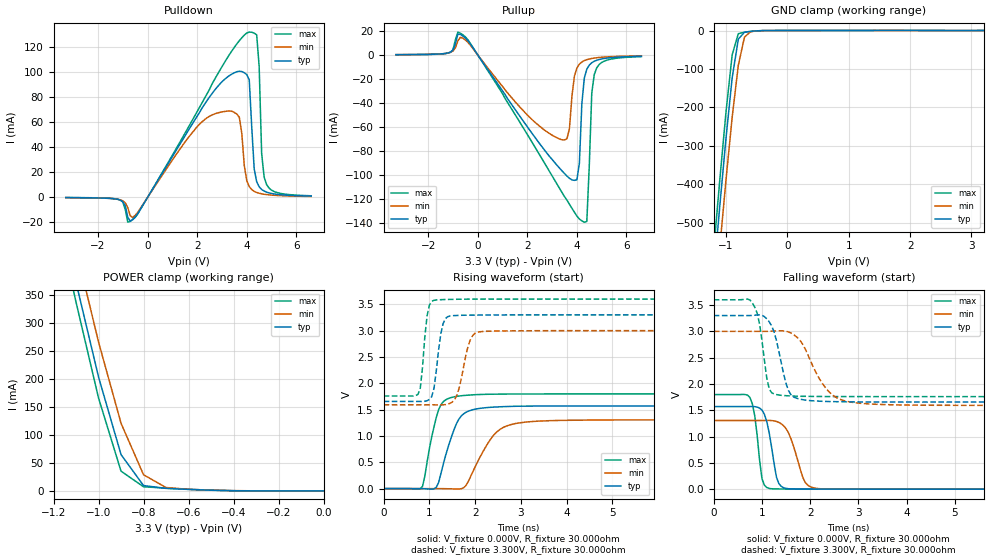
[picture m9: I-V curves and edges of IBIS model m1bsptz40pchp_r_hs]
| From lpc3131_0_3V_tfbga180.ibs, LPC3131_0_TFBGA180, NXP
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| |   Rev 0.20 IBIS Model Design Automation Generation   |
| |   N O N - S I L I C O N   C O R R E L A T E D   |
| |   This IBIS [Model] is pre-Beta tactical support   |
| |  Note: this IBIS [Model] contains clamp curves generated   |
| |   through simulation which should not be relied upon   |
| Date/Time   : 2010 Jan 25 (Mon) 11:58:19
| Pccmos090 jliolib_p50 2.0
|   0.9 um 3.3V pad library
|   seven level metal
|   dual oxide
|   dual threshold voltage
|   nominal line mixed supply
|   parasitic extracted netlists
| Process block a10
| mem1bsptz40pchp
|   Bidirectional Pad 3.3
|   3state Output
|   Plain Input
|   CMOS
|   Programmable between
|   - (p1=0, p2=1) plain input
|   - (p1=0, p2=0) with Pull Up
|   - (p1=1, p2=1) with Pull Down
|   - (p1=1, p2=0) with Repeater
| Repeater Mode high speed(esh=0, p1=1, p2=0)
[Model]   m1bsptz40pchp_r_hs | of mem1bsptz40pchp
Model_type   I/O
Polarity   Non-Inverting
Enable   Active-Low
|  Reciever Thresholds
Vinl   = 0.99V
Vinh   = 2.31V
| AC Test Load Conditions
Vref   = 0
Cref   = 0
Rref   = 1000000000
Vmeas   = 1.65
| [Process Range]   typical   min   max
| C_comp edge width   400.000ps   400.000ps   400.000ps
| C_comp Tstrobe   40.000fs   40.000fs   40.000fs
C_comp   200.000pF   200.000pF   200.000pF
[Temperature Range]   25   125   -40
[Voltage Range]   3.30V   3.00V   3.60V
[GND Clamp Reference]   0.00V   0.00V   0.00V
[Pulldown Reference]   0.00V   0.00V   0.00V
[POWER Clamp Reference]   3.30V   3.00V   3.60V
[Pullup Reference]   3.30V   3.00V   3.60V
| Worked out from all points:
|   slope of the pulldown table from 0 to 0.495 V, typ, clamps not added: 30.9 ohm
|   slope of the pullup table from 0 to 0.495 V, typ, clamps not added: 33.4 ohm
|   GND clamp passes 1 mA (typ) near -0.51 V on its own axis
|   POWER clamp passes 1 mA (typ) near -0.47 V on its own axis
|   rising waveform, V_fixture 0.000V, R_fixture 30.000ohm: 20-80 % time 345ps typ, 518ps min, 258ps max; typ from 0 V to 1.57 V
|   falling waveform, V_fixture 0.000V, R_fixture 30.000ohm: 20-80 % time 178ps typ, 273ps min, 137ps max; typ from 1.57 V to 0 V
|   rising waveform, V_fixture 3.300V, R_fixture 30.000ohm: 20-80 % time 145ps typ, 213ps min, 116ps max; typ from 1.66 V to 3.3 V
|   falling waveform, V_fixture 3.300V, R_fixture 30.000ohm: 20-80 % time 251ps typ, 503ps min, 170ps max; typ from 3.3 V to 1.66 V
[GND Clamp]
| ref voltage   0.00V   0.00V   0.00V
|   Voltage   I(typ)   I(min)   I(max)
-3.3V     -4.732A    -4.814A    -4.684A
-1.2V     -636mA     -742.5mA   -569.7mA
-1.1V     -453.5mA   -561.8mA   -385.7mA
-1V       -279mA     -387.5mA   -210.8mA
-900mV    -122.8mA   -225.5mA   -63.13mA
-800mV    -22.45mA   -90.49mA   -8.204mA
-700mV    -4.394mA   -17.31mA   -4.534mA
-600mV    -2.163mA   -3.055mA   -2.529mA
-300mV    -78.17uA   -69.01uA   -98.11uA
3.2V      -17.82uA   34.39uA    -87.56uA
[Power Clamp]   | Vtable = Vcc - Vpad
| ref voltage   3.30V   3.00V   3.60V
|   Voltage   I(typ)   I(min)   I(max)
-3.3V     4.647A     4.675A     4.636A
-1.2V     553.3mA    610.4mA    520.8mA
-1.1V     373.2mA    433.6mA    337.9mA
-1V       204mA      266.6mA    166.4mA
-900mV    65.07mA    121.2mA    35.4mA
-800mV    9.632mA    28.93mA    7.456mA
-700mV    4.576mA    6.079mA    4.901mA
-600mV    2.711mA    2.826mA    2.897mA
-400mV    366.5uA    549.1uA    304.5uA
0V        388.1pA    9.875nA    264.4pA
[Pulldown]
| ref voltage   0.00V   0.00V   0.00V
|   Voltage   I(typ)   I(min)   I(max)
-3.3V     -236.7uA   -252.6uA   -192uA
-1.2V     -1.652mA   -1.556mA   -1.496mA
-600mV    -17.54mA   -16.01mA   -17.75mA
2.9V      89.88mA    67.56mA    100.6mA
3.7V      100.4mA    63.73mA    124.7mA
4.1V      93.46mA    8.514mA    131.5mA
4.3V      22.53mA    4.741mA    130.7mA
4.4V      12.45mA    3.859mA    129.3mA
4.5V      8.406mA    3.243mA    104mA
4.6V      6.249mA    2.791mA    34.96mA
4.8V      4.128mA    2.175mA    10.1mA
6.6V      975.1uA    710.1uA    1.222mA
[Pullup]   | Vtable = Vcc - Vpad
| ref voltage   3.30V   3.00V   3.60V
|   Voltage   I(typ)   I(min)   I(max)
-3.3V     206.8uA    209.1uA    174.1uA
-500mV    14.05mA    12.42mA    15mA
3.4V      -96.32mA   -70.52mA   -114.2mA
3.7V      -102.5mA   -61.11mA   -124.1mA
3.9V      -104.2mA   -17.59mA   -130.7mA
4.1V      -89.97mA   -7.665mA   -136.3mA
4.2V      -40.47mA   -5.865mA   -137.9mA
4.3V      -19.14mA   -4.724mA   -138.9mA
4.4V      -11.89mA   -3.942mA   -138.3mA
4.6V      -6.502mA   -2.948mA   -31.69mA
4.7V      -5.28mA    -2.614mA   -16.33mA
6.6V      -1.118mA   -810uA     -1.413mA
[Ramp]
R_load   = 30.000ohm
|   dV/dt(typ)   dV/dt(min)   dV/dt(max)
dV/dt_r   941.960mV/350.000ps   783.290mV/500.000ps   1.079V/250.000ps
dV/dt_f   986.686mV/250.000ps   845.150mV/500.000ps   1.104V/150.000ps
[Rising Waveform]  | cubic spline decimation from 501 points
V_fixture   = 0.000V
R_fixture   = 30.000ohm
|   Time   V(typ)   V(min)   V(max)
0s        3.993nV    181.6nV    2.818nV
850ps     -1.566mV   23.17uV    44.27mV
1.15ns    23.74mV    142.8uV    1.35V
1.35ns    615.7mV    -1.771mV   1.683V
1.6ns     1.249V     -8.251mV   1.752V
1.75ns    1.422V     16.92mV    1.769V
2.45ns    1.55V      1.058V     1.794V
2.75ns    1.56V      1.208V     1.796V
3.35ns    1.568V     1.28V      1.797V
25ns      1.57V      1.305V     1.798V
[Falling Waveform]  | cubic spline decimation from 501 points
V_fixture   = 0.000V
R_fixture   = 30.000ohm
|   Time   V(typ)   V(min)   V(max)
0s        1.57V      1.305V     1.798V
750ps     1.571V     1.305V     1.742V
850ps     1.569V     1.305V     1.395V
1ns       1.504V     1.306V     198.2mV
1.2ns     794.7mV    1.304V     7.889mV
1.3ns     230.7mV    1.287V     5.056mV
1.4ns     53.05mV    1.243V     3.511mV
1.9ns     2.347mV    124.6mV    939.1uV
2.2ns     1.383mV    8.421mV    234.7uV
25ns      7.487nV    232.3nV    70.99nV
[Rising Waveform]  | cubic spline decimation from 501 points
V_fixture   = 3.300V
V_fixture_min = 3.000V
V_fixture_max = 3.600V
R_fixture   = 30.000ohm
|   Time   V(typ)   V(min)   V(max)
0s        1.656V     1.591V     1.759V
750ps     1.655V     1.591V     1.791V
800ps     1.655V     1.591V     1.903V
950ps     1.67V      1.591V     3.285V
1.15ns    2.234V     1.59V      3.583V
1.35ns    3.229V     1.596V     3.592V
1.6ns     3.288V     1.772V     3.596V
1.9ns     3.295V     2.84V      3.599V
2.2ns     3.298V     2.986V     3.599V
25ns      3.3V       3V         3.6V
[Falling Waveform]  | cubic spline decimation from 501 points
V_fixture   = 3.300V
V_fixture_min = 3.000V
V_fixture_max = 3.600V
R_fixture   = 30.000ohm
|   Time   V(typ)   V(min)   V(max)
0s        3.3V       3V         3.6V
800ps     3.303V     3V         3.54V
950ps     3.313V     3V         3.141V
1.15ns    3.181V     3.002V     1.906V
1.25ns    2.993V     3.006V     1.81V
1.45ns    2.188V     3.009V     1.78V
1.7ns     1.735V     2.908V     1.768V
2.4ns     1.666V     1.842V     1.761V
3.1ns     1.658V     1.628V     1.76V
25ns      1.656V     1.591V     1.759V
